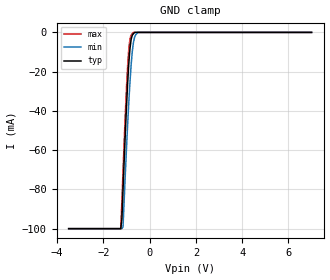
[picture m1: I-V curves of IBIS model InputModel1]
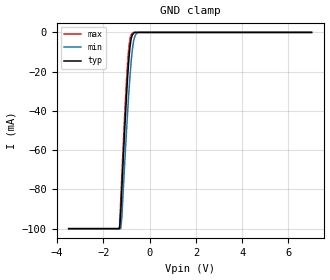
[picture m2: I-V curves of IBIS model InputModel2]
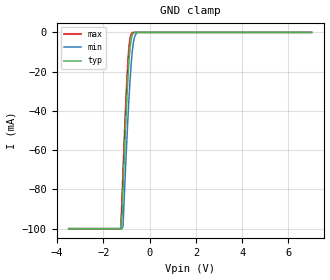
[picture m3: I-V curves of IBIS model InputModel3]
[IBIS Ver]   2.1
[File name]   e008sal3.ibs  | e_= TSOP, f0008sa-l= abbr chip name, 3=3.3V Vcc
[File Rev]   2.00
[Date]   3-April-96
[Source]   File generated from lab measurements at Intel Corporation
[Notes]   Rev 2.00 All data was replaced by actual measurements
   performed in a lab.
[Disclaimer] INTEL DEVELOPER'S SOFTWARE LICENSE AGREEMENT
| BY USING THIS SOFTWARE, YOU ARE AGREEING TO BE BOUND
| BY THE TERMS OF THIS AGREEMENT.  DO NOT USE THE SOFTWARE
| UNTIL YOU HAVE CAREFULLY READ AND AGREED TO THE FOLLOWING
| TERMS AND CONDITIONS.  IF YOU DO NOT AGREE TO THE TERMS
| OF THIS AGREEMENT, PROMPTLY RETURN THE SOFTWARE PACKAGE
| AND ANY ACCOMPANYING ITEMS.
| IF YOU USE THIS SOFTWARE, YOU WILL BE BOUND BY THE TERMS
| OF THIS AGREEMENT
| LICENSE: Intel Corporation ("Intel") grants you the non-exclusive right
| to use the enclosed software program ("Software").  You will not use,
| copy, modify, rent, sell or transfer the Software or any portion
| thereof, except as provided in this Agreement.
| System OEM Developers may:
| 1.   Copy the Software for support, backup or archival purposes;
| 2.   Install, use, or distribute Intel owned Software in object code
|   only;
| 3.   Modify and/or use Software source code that Intel directly makes
|   available to you as an OEM Developer;
| 4.   Install, use, modify, distribute, and/or make or have made
|   derivatives ("Derivatives") of Intel owned Software under the
|   terms and conditions in this Agreement, ONLY if you are a System
|   OEM Developer and NOT an end-user.
| RESTRICTIONS:
| YOU WILL NOT:
| 1.   Copy the Software, in whole or in part, except as provided for
|   in this Agreement;
| 2.   Decompile or reverse engineer any Software provided in object
|   code format;
| 3.   Distribute any Software or Derivative code to any end-users,
|   unless approved by Intel in a prior writing.
| TRANSFER: You may transfer the Software to another OEM
| Developer if the receiving party agrees to the terms of this
| Agreement at the sole risk of any receiving party.
| OWNERSHIP AND COPYRIGHT OF SOFTWARE:
| Title to the Software and all copies thereof remain with Intel
| or its vendors.  The Software is copyrighted and is protected by
| United States and international copyright laws.  You will not
| remove the copyright notice from the Software.  You agree to
| prevent any unauthorized copying of the Software.
| DERIVATIVE WORK: OEM Developers that make or have made
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[Copyright]   Copyright 1996, Intel Corporation, All Rights Reserved
[Component]   E28F008SA-L   | 40-lead TSOP package, 28F008SA-L
[Manufacturer]  Intel   | Flash File (tm)
|   | operating in 3.3 V Vcc range
[Package]
|The following values apply for the leadframe.
|Variable   typ   min   max
R_pkg   135m   126m   144m
L_pkg   3.95nH   3.62nH   4.28nH
C_pkg   0.39pF   0.38pF   0.40pF
|*****************************Pin Definitions**********************************
[Pin]   signal_name   model_name   R_pin   L_pin   C_pin
  1   A19   InputModel2
  2   A18   InputModel2
  3   A17   InputModel2
  4   A16   InputModel2
  5   A15   InputModel2
  6   A14   InputModel2
  7   A13   InputModel2
  8   A12   InputModel2
  9   CE#   InputModel3
 10   VCC   POWER
 11   VPP   POWER
 12   RP#   InputModel4
 13   A11   InputModel2
 14   A10   InputModel2
 15   A09   InputModel2
 16   A08   InputModel2
 17   A07   InputModel2
 18   A06   InputModel2
 19   A05   InputModel2
 20   A04   InputModel2
 21   A03   InputModel1
 22   A02   InputModel1
 23   A01   InputModel1
 24   A00   InputModel1
 25   DQ0   InputOutput
 26   DQ1   InputOutput
 27   DQ2   InputOutput
 28   DQ3   InputOutput
 29   GND   GND
 30   GND   GND
 31   VCC   POWER
 32   DQ4   InputOutput
 33   DQ5   InputOutput
 34   DQ6   InputOutput
 35   DQ7   InputOutput
 36   RY/BY#   RYBYOutput
 37   OE#   InputModel3
 38   WE#   InputModel3
 39   NC   InputModel5
 40   NC   InputModel5
|**********************Input Model 5***************************************
[Model]   InputModel5
Model_type   Input
|   For NC pins
Vinl = 0.8V
Vinh = 2.0V
| Variable   typ   min   max
C_comp   5.61p   NA   7.6p
[Voltage Range]   3.3V   3.0V   3.6V
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| Models and submodels in the file (7): InputModel1 (Input), InputModel2 (Input), InputModel3 (Input), InputModel4 (Input), InputModel5 (Input), InputOutput (I/O), RYBYOutput (Output)
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|**************************Input Model 1***************************************
[Model]   InputModel1
Model_type   Input
|   For A[3:0]
Vinl = 0.8V
Vinh = 2.0V
| Variable   typ   min   max
C_comp   5.61p   NA   7.6p
[Voltage Range]   3.3V   3.0V   3.6V
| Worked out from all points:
|   GND clamp passes 1 mA (typ) near -0.72 V on its own axis
[GND_clamp]
|Voltage I(typ)   I(min)   I(max)
-3.5V     -100mA     -100mA     -100mA
-1.25V    -100mA     -100mA     -100mA
-1.2V     -95.07mA   -100mA     -86.07mA
-1.15V    -79.86mA   -99mA      -70.4mA
-1.05V    -50.95mA   -71.8mA    -41.05mA
-950mV    -25.72mA   -46.61mA   -16.75mA
-900mV    -15.57mA   -35.21mA   -8.231mA
-850mV    -8.181mA   -25.25mA   -3.35mA
-800mV    -3.515mA   -16.43mA   -1.299mA
-700mV    -671.7uA   -5.073mA   0A
-500mV    0A         0A         0A
7V        0A         0A         0A
[POWER_clamp]
| Input buffer circuits of this product do not intrinsically
| require a [POWER_clamp] definition.  This zero current
| [POWER_clamp] is provided for compatibility with some ibis
| parsers.
|Voltage  I(typ)   I(min)   I(max)
-3.3V     0A         0A         0A
0V        0A         0A         0A
3.3V      0A         0A         0A
6.6V      0A         0A         0A
|**********************Input Model 2************************************
[Model]   InputModel2
Model_type   Input
|   For A[19:4]
Vinl = 0.8V
Vinh = 2.0V
| Variable   typ   min   max
C_comp   5.61p   NA   7.6p
[Voltage Range]   3.3V   3.0V   3.6V
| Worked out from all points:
|   GND clamp passes 1 mA (typ) near -0.73 V on its own axis
[GND_clamp]
|Voltage I(typ)   I(min)   I(max)
-3.5V     -100mA     -100mA     -100mA
-1.3V     -100mA     -100mA     -99.05mA
-1.25V    -91.91mA   -100mA     -85.56mA
-1.2V     -79.19mA   -94.07mA   -72.29mA
-1.05V    -43.33mA   -60.73mA   -35.37mA
-950mV    -22.48mA   -40.12mA   -14.99mA
-900mV    -13.9mA    -30.69mA   -7.576mA
-850mV    -7.472mA   -22.37mA   -3.135mA
-800mV    -3.262mA   -14.88mA   -1.175mA
-700mV    -582uA     -4.802mA   0A
-500mV    0A         0A         0A
7V        0A         0A         0A
[POWER_clamp]
| Input buffer circuits of this product do not intrinsically
| require a [POWER_clamp] definition.  This zero current
| [POWER_clamp] is provided for compatibility with some ibis
| parsers.
|Voltage  I(typ)   I(min)   I(max)
-3.3V     0A         0A         0A
0V        0A         0A         0A
3.3V      0A         0A         0A
6.6V      0A         0A         0A
|*********************Input Model 3**************************************
[Model]   InputModel3
Model_type   Input
|   For WE#, OE# & CE#
Vinl = 0.8V
Vinh = 2.0V
| Variable   typ   min   max
C_comp   5.61p   NA   7.6p
[Voltage Range]   3.3V   3.0V   3.6V
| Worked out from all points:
|   GND clamp passes 1 mA (typ) near -0.74 V on its own axis
[GND_clamp]
|Voltage I(typ)   I(min)   I(max)
-3.5V     -100mA     -100mA     -100mA
-1.25V    -100mA     -100mA     -100mA
-1.2V     -95.1mA    -100mA     -86.12mA
-1.15V    -79.72mA   -98.88mA   -70.26mA
-1.05V    -50.65mA   -71.61mA   -40.78mA
-950mV    -25.39mA   -46.36mA   -16.47mA
-900mV    -15.22mA   -34.94mA   -7.948mA
-850mV    -7.856mA   -24.98mA   -3.051mA
-750mV    -1.172mA   -9.488mA   0A
-650mV    0A         -2.268mA   0A
-550mV    0A         0A         0A
7V        0A         0A         0A
[POWER_clamp]
| Input buffer circuits of this product do not intrinsically
| require a [POWER_clamp] definition.  This zero current
| [POWER_clamp] is provided for compatibility with some ibis
| parsers.
|Voltage  I(typ)   I(min)   I(max)
-3.3V     0A         0A         0A
0V        0A         0A         0A
3.3V      0A         0A         0A
6.6V      0A         0A         0A
